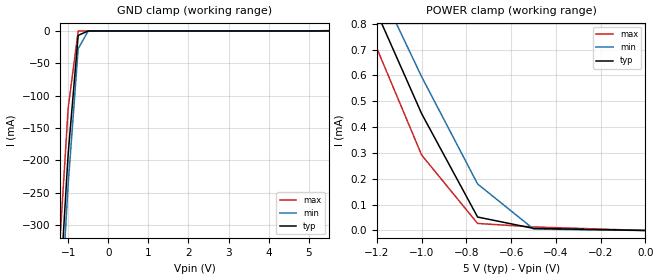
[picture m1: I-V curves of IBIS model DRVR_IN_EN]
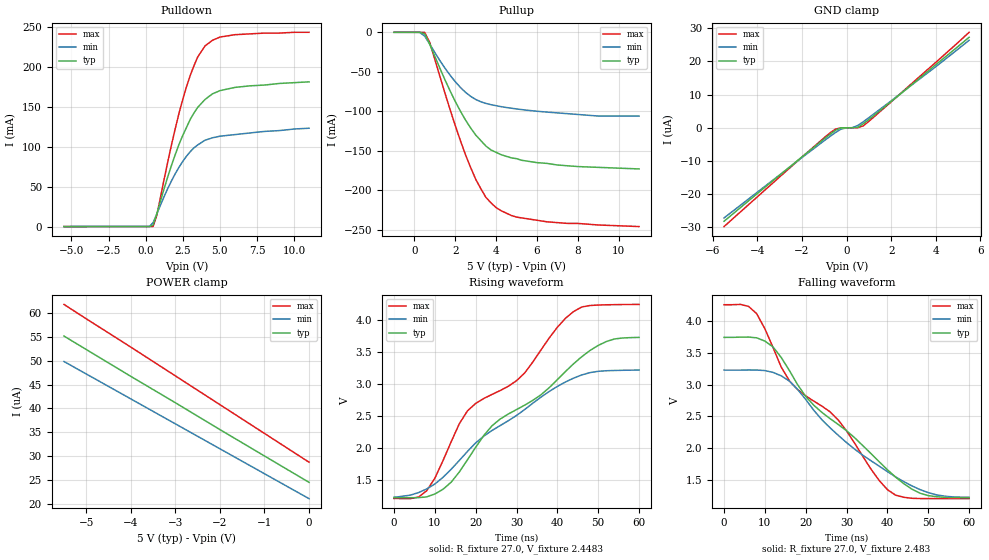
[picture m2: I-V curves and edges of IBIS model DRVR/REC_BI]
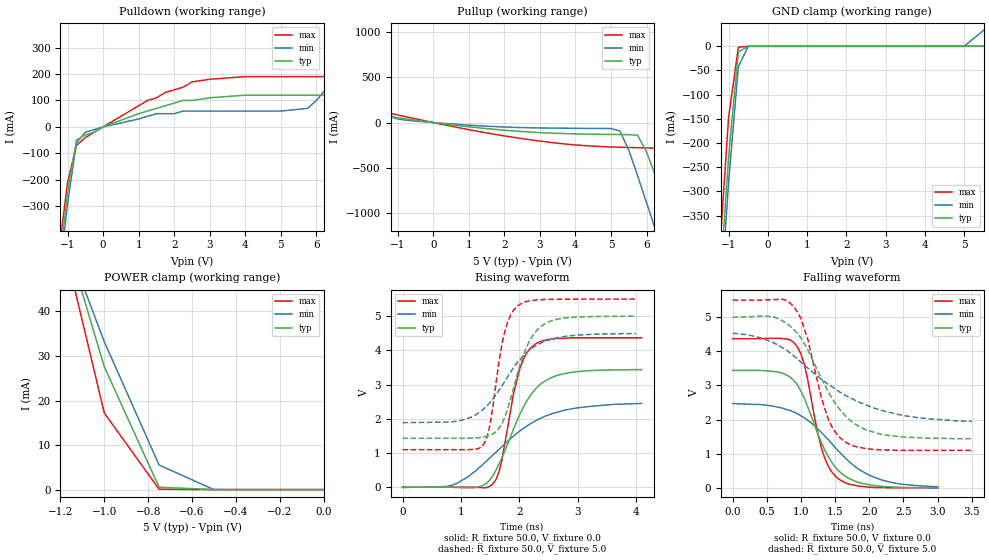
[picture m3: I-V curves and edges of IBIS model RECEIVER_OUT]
|   Texas Instruments Incorporated
|   Data Transmissions Products
|   IBIS Model for SN65HVD24
|   8D SOIC Package
[IBIS Ver]   3.2
[Comment char]   |_char
[File name]   sllc159a.ibs
[File Rev]   1.0
[Date]   19Jun03
[Source]   File originated at Texas Instruments Incorporated.
   Data Transmission Products Group.
[Notes]
[Disclaimer]
(C) Copyright Texas Instruments Incorporated 2003
   All rights reserved
  Texas Instruments Incorporated hereby grants the user of this IBIS
model a non-exclusive, nontransferable license to use this IBIS model
under the following terms.  Before using this IBIS model, the user
should read this license.  If the user does not accept these terms,
the IBIS model should be returned to Texas Instruments within 30 days.
  The user is granted this license only to use the IBIS model and
is not granted rights to sell, load, rent, lease or license the IBIS
model in whole or in part, or in modified form to anyone other than
user.  User may modify the IBIS model to suit its specific applications
but rights to derivative works and such modifications shall belong to
Texas Instruments.
  This IBIS model is provided on an "AS IS" basis and Texas Instruments
makes absolutely no warranty with respect to the information contained
herein.  TEXAS INSTRUMENTS DISCLAIMS AND CUSTOMER WAIVES ALL WARRANTIES,
EXPRESS OR IMPLIED, INCLUDING WARRANTIES OF MERCHANTABILITY OR FITNESS
FOR A PARTICULAR PURPOSE. The entire risk as to quality and performance
is with the Customer. ACCORDINGLY, IN NO EVENT SHALL THE COMPANY BE LIABLE
FOR ANY DAMAGES, WHETHER IN CONTRACT OR TORT,INCLUDING ANY LOST PROFITS
OR OTHER INCIDENTAL, CONSEQUENTIAL, EXEMPLARY, OR PUNITIVE DAMAGES ARISING
OUT OF THE USE OR APPLICATION OF THE IBIS model provided in this package.
Further, Texas Instruments reserves the right to discontinue or make changes
without notice to any product herein to improve reliability, function, or
design. Texas Instruments does not convey any license under patent rights
or any other intellectual property rights, including those of third parties.
Contact Texas Instruments at ATTN:DATA TRANSMISSIONS
[Copyright]   Copyright 2003, Texas Instruments, All Rights Reserved
[Component]   HVD24D
[Manufacturer]  Texas Instruments Incorporated
[Package]
|   typ   min   max
R_pkg   0.055   0.034   0.067
L_pkg   1.795nH   1.699nH   1.914nH
C_pkg   0.299pF   0.278pF   0.311pF
[Pin]   signal_name   model_name   R_pin   L_pin   C_pin
1   R   RECEIVER_OUT   0.067   1.914n   0.278p
2   RE   DRVR_IN_EN   0.062   1.816n   0.301p
3   DE   DRVR_IN_EN   0.053   1.699n   0.298p
4   D   DRVR_IN_EN   0.067   1.907n   0.278p
5   GND   GND   0.034   1.704n   0.311p
6   A   DRVR/REC_BI   0.061   1.808n   0.310p
7   B   DRVR/REC_BI   0.062   1.817n   0.302p
8   VCC   POWER   0.034   1.716n   0.311p
[Diff_pin]   inv_pin   vdiff   tdelay_typ   tdelay_min   tdelay_max
| The 'A' pin is Diff_pin and the 'B' pin is the inv_pin
6   7   0.200   0 0 0
| Models and submodels in the file (3): DRVR_IN_EN (Input), DRVR/REC_BI (I/O), RECEIVER_OUT (3-state)
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|   Driver Input / Receiver Enable Model
[Model]   DRVR_IN_EN
Model_type   Input
|Signals   D,DE,RE
Vinh = 2.0
Vinl = 0.8
|   typ   min   max
C_comp   1.0pF   NA   NA
|   typ   min   max
[Temperature Range]   25.0   -40   125
[Voltage range]   5.0V   4.5V   5.5V
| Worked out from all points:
|   GND clamp passes 1 mA (typ) near -0.54 V on its own axis
|   POWER clamp passes 1 mA (typ) near -1.28 V on its own axis
[GND_clamp]
|   Voltage   I(typ)   I(min)   I(max)
-5.5V     -4.7A      -4.83A     -4.52A
-2V       -1.22A     -1.29A     -1.12A
-1V       -190mA     -237mA     -119mA
-750mV    -6.83mA    -27.3mA    -170uA
-500mV    -28.3uA    -38.2uA    -58.3uA
5.5V      8.09uA     595uA      14.3pA
[Power_clamp]
| Note that the[POWER_clamp]voltage table is referenced to Vcc
| and is calculated using Vtable=Vcc - Vmeasured.
|   Voltage   I(typ)   I(min)   I(max)
-5.5V     9.83mA     9.25mA     10.5mA
-1.25V    941uA      1.05mA     808uA
-1V       452uA      595uA      292uA
-750mV    52uA       180uA      27.1uA
-500mV    8.09uA     5.88uA     13.7uA
0V        0A         0A         0A
|   Driver Output / Receiver Input Model
[Model]   DRVR/REC_BI
Model_type   I/O
| Signals   A,B
Vinl = 0.9V
Vinh = 2.8V
Vmeas = 1.7V   |Reference voltage for timing measurements
Cref = 50pF   |Timing specification test load capacitance value
Rref = 54   |Note: 54 Ohm load; single-ended configuration
|   Timing specification test load voltage
| variable   typ   min   max
C_comp   1.0pF   NA   NA
|   typ   min   max
[Temperature Range]   25.0   -40   85
[Voltage range]   5.0V   4.5V   5.5V
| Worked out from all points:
|   slope of the pulldown table from 0 to 0.75 V, typ, clamps not added: 47.1 ohm
|   slope of the pullup table from 0 to 0.75 V, typ, clamps not added: 49.5 ohm
|   rising waveform, R_fixture 27.0, V_fixture 2.4483: 20-80 % time 25.5ns typ, 23.2ns min, 25ns max; typ from 1.23 V to 3.73 V
|   falling waveform, R_fixture 27.0, V_fixture 2.483: 20-80 % time 23.1ns typ, 20.9ns min, 23ns max; typ from 3.74 V to 1.23 V
[Pulldown]
|   Voltage   I(typ)   I(min)   I(max)
-5.5V     -47.3uA    -37.5uA    -52.8uA
250mV     -13.8uA    29.6uA     -17uA
500mV     1.9mA      4.84mA     48.4uA
750mV     15.9mA     15.6mA     13.8mA
1.75V     77.1mA     57.5mA     103mA
2.5V      114mA      81.5mA     159mA
3.25V     142mA      98.4mA     201mA
3.5V      149mA      102mA      212mA
4V        159mA      108mA      226mA
5V        170mA      113mA      237mA
6V        174mA      115mA      240mA
11V       181mA      123mA      243mA
[Pullup]
|   Voltage   I(typ)   I(min)   I(max)
| Note that the[Pullup]voltage table is referenced to Vcc
| and is calculated using Vtable=Vcc - Vmeasured.
-1V       78uA       65.4uA     90.8uA
250mV     57.2uA     6.09uA     70uA
500mV     -1.82mA    -4.63mA    1.15uA
750mV     -15.1mA    -14.9mA    -12.9mA
1.75V     -74.3mA    -54.4mA    -98.1mA
2.25V     -99.7mA    -69.7mA    -137mA
2.75V     -121mA     -81mA      -171mA
3.5V      -144mA     -90mA      -209mA
4V        -152mA     -92.9mA    -222mA
5V        -160mA     -97mA      -234mA
6.5V      -166mA     -101mA     -240mA
11V       -173mA     -106mA     -246mA
[GND_clamp]
|   Voltage   I(typ)   I(min)   I(max)
| Outputs in High Impedance (off)
-5.5V     -28.2uA    -27.2uA    -29.8uA
-2V       -8.77uA    -8.98uA    -8.83uA
-750mV    -2.01uA    -2.64uA    -1.6uA
-500mV    -761nA     -1.45uA    -411nA
-250mV    -19.5nA    -417nA     -9.75nA
0V        -3.7nA     -3.55nA    -3.96nA
250mV     -3.11nA    22.2nA     -3.43nA
500mV     129nA      679nA      -2.68nA
750mV     1.2uA      1.82uA     578nA
4V        19uA       18.4uA     19.7uA
5.5V      27.3uA     26.4uA     28.8uA
[POWER_clamp]
|   Voltage   I(typ)   I(min)   I(max)
| Note that the [POWER_clamp] voltage table is referenced to Vcc
| and is calculated using Vtable = Vcc - Vmeasured.
| Outputs in Tri-state.
-5.5V     55.1uA     49.8uA     61.7uA
-5V       52.3uA     47.2uA     58.7uA
-4V       46.7uA     42uA       52.8uA
-3V       41.2uA     36.8uA     46.8uA
-2V       35.6uA     31.6uA     40.8uA
-1V       30.1uA     26.4uA     34.8uA
0V        24.6uA     21.2uA     28.8uA
[Ramp]
|   typ   min   max
dV/dt_r   1.50V/25.4ns   1.20V/22.6ns   1.82V/25.0ns
dV/dt_f   1.51V/23.1ns   1.20V/20.9ns   1.82V/23.0ns
R_load = 27ohm | Note: The measurement is on a single-ended configuration
|   with 54ohm line-to-line.
[Rising Waveform]
R_fixture = 27.0
V_fixture = 2.4483
V_fixture_min = 2.227
V_fixture_max = 2.73
C_fixture = 0p
L_fixture = 0n
|   V(typ)   V(min)   V(max)
0s        1.226V     1.228V     1.211V
8ns       1.236V     1.36V      1.331V
12ns      1.355V     1.542V     1.803V
18ns      1.817V     1.948V     2.582V
24ns      2.348V     2.274V     2.838V
30ns      2.601V     2.509V     3.052V
36ns      2.833V     2.796V     3.535V
44ns      3.319V     3.093V     4.135V
52ns      3.665V     3.208V     4.239V
60ns      3.729V     3.219V     4.245V
[Falling Waveform]
R_fixture = 27.0
V_fixture = 2.483
V_fixture_min = 2.227
V_fixture_max = 2.73
C_fixture = 0p
L_fixture = 0n
|   V(typ)   V(min)   V(max)
0s        3.74V      3.227V     4.252V
6ns       3.745V     3.229V     4.226V
8ns       3.733V     3.228V     4.111V
12ns      3.59V      3.191V     3.582V
16ns      3.221V     3.055V     3.06V
22ns      2.675V     2.595V     2.74V
28ns      2.373V     2.203V     2.443V
40ns      1.665V     1.636V     1.353V
48ns      1.297V     1.354V     1.214V
60ns      1.229V     1.232V     1.212V
|   Receiver Output Model
[Model]   RECEIVER_OUT
Model_type   3-state
| Signals   R
Vmeas = 2.2V   |Reference voltage for timing measurements
Cref = 15pF   |Timing specification test load capacitance value
Vref = 0   |Timing specification test load voltage; GND
| variable   typ   min   max
C_comp   1.0pF   NA   NA
|   typ   min   max
[Temperature Range]   25.0   -40   85
[Voltage range]   5.0V   4.5V   5.5V
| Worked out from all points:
|   slope of the pulldown table from 0 to 0.75 V, typ, clamps not added: 20 ohm
|   slope of the pullup table from 0 to 0.75 V, typ, clamps not added: 21 ohm
|   GND clamp passes 1 mA (typ) near -0.52 V on its own axis
|   POWER clamp passes 1 mA (typ) near -0.75 V on its own axis
|   rising waveform, R_fixture 50.0, V_fixture 0.0: 20-80 % time 566ps typ, 1.04ns min, 306ps max; typ from 0 V to 3.44 V
|   falling waveform, R_fixture 50.0, V_fixture 0.0: 20-80 % time 454ps typ, 770ps min, 285ps max; typ from 3.44 V to 0 V
|   rising waveform, R_fixture 50.0, V_fixture 5.0: 20-80 % time 409ps typ, 689ps min, 252ps max; typ from 1.43 V to 5 V
|   falling waveform, R_fixture 50.0, V_fixture 5.0: 20-80 % time 602ps typ, 1.1ns min, 351ps max; typ from 5 V to 1.44 V
[Pulldown]
|   Voltage   I(typ)   I(min)   I(max)
-5.5V     -5.53A     -5.49A     -5.57A
-1.25V    -540mA     -580mA     -480mA
-1V       -250mA     -290mA     -210mA
-750mV    -50mA      -60mA      -70mA
-500mV    -30mA      -20mA      -40mA
1.25V     60mA       40mA       100mA
2.5V      100mA      60mA       170mA
5.75V     120mA      70mA       190mA
6.5V      130mA      170mA      190mA
7.25V     250mA      270mA      200mA
8V        380mA      380mA      360mA
11V       920mA      800mA      1.05A
[Pullup]
|   Voltage   I(typ)   I(min)   I(max)
| Note that the[Pullup]voltage table is referenced to Vcc
| and is calculated using Vtable=Vcc - Vmeasured.
-5.5V     831mA      660mA      1.05A
-1.5V     116mA      101mA      135mA
-750mV    38.6mA     25.2mA     62.6mA
1.5V      -66.6mA    -39.9mA    -114mA
5.25V     -132mA     -93mA      -272mA
5.75V     -140mA     -586mA     -277mA
6V        -324mA     -882mA     -279mA
6.25V     -583mA     -1.18A     -282mA
6.5V      -849mA     -1.47A     -402mA
7V        -1.44A     -2.06A     -909mA
8V        -2.62A     -3.21A     -1.99A
11V       -6.03A     -6.64A     -5.58A
[GND_clamp]
|   Voltage   I(typ)   I(min)   I(max)
| Outputs in High Impedance (off)
-5.5V     -5.53A     -5.49A     -5.57A
-1.25V    -531mA     -579mA     -452mA
-1V       -230mA     -282mA     -148mA
-750mV    -11.8mA    -42mA      -2.02mA
-500mV    -7.54uA    -155uA     -41.3uA
5V        0A         5.88uA     -7.45nA
5.5V      22.4nA     33.2mA     -7.45nA
[POWER_clamp]
|   Voltage   I(typ)   I(min)   I(max)
| Note that the [POWER_clamp] voltage table is referenced to Vcc
| and is calculated using Vtable = Vcc - Vmeasured.
| Outputs in Tri-state.
-5.5V     845mA      659mA      1.05A
-1.25V    68.8mA     65.7mA     68.8mA
-1V       27.6mA     33.2mA     17.2mA
-750mV    537uA      5.52mA     88.4uA
-500mV    22.4nA     5.88uA     0A
0V        0A         0A         -7.45nA
[Ramp]
|   typ   min   max
dV/dt_r   2.06V/563ns   1.47V/1038ps   2.62V/306ps
dV/dt_f   2.14V/599ps   1.55V/1103ps   2.64V/346ps
R_load = 50
[Rising Waveform]
R_fixture = 50.0
V_fixture = 0.0
C_fixture = 0p
L_fixture = 0n
|   V(typ)   V(min)   V(max)
0s        0V         -10mV      0V
900ps     -10mV      90mV       0V
1.35ns    30mV       620mV      -10mV
1.55ns    340mV      940mV      100mV
1.7ns     840mV      1.18V      760mV
1.9ns     1.69V      1.49V      2.71V
2ns       2.09V      1.63V      3.41V
2.3ns     2.91V      1.96V      4.21V
2.9ns     3.36V      2.29V      4.37V
4.1ns     3.44V      2.45V      4.37V
[Falling Waveform]
R_fixture = 50.0
V_fixture = 0.0
C_fixture = 0p
L_fixture = 0n
|   V(typ)   V(min)   V(max)
0s        3.44V      2.47V      4.37V
700ps     3.38V      2.35V      4.38V
950ps     3.01V      2.17V      4.12V
1.05ns    2.62V      2.05V      3.61V
1.3ns     1.32V      1.62V      1.16V
1.4ns     910mV      1.41V      630mV
1.55ns    500mV      1.07V      260mV
1.8ns     190mV      610mV      70mV
2.1ns     60mV       290mV      10mV
3ns       0V         30mV       0V
[Rising Waveform]
R_fixture = 50.0
V_fixture = 5.0
V_fixture_min = 4.5
V_fixture_max = 5.5
C_fixture = 0p
L_fixture = 0n
|   V(typ)   V(min)   V(max)
0s        1.43V      1.887V     1.097V
950ps     1.428V     1.938V     1.096V
1.4ns     1.472V     2.302V     1.276V
1.5ns     1.519V     2.481V     1.827V
1.65ns    1.709V     2.822V     3.631V
1.75ns    2.037V     3.084V     4.53V
2ns       3.497V     3.713V     5.336V
2.2ns     4.345V     4.039V     5.456V
2.5ns     4.831V     4.303V     5.492V
4ns       4.999V     4.493V     5.5V
[Falling Waveform]
R_fixture = 50.0
V_fixture = 5.0
V_fixture_min = 4.5
V_fixture_max = 5.5
C_fixture = 0p
L_fixture = 0n
|   V(typ)   V(min)   V(max)
0s        5V         4.53V      5.5V
600ps     5.01V      4.25V      5.52V
900ps     4.63V      3.86V      5.29V
1ns       4.39V      3.68V      4.96V
1.1ns     4.04V      3.51V      4.35V
1.3ns     3.2V       3.18V      2.63V
1.4ns     2.81V      3.03V      2.01V
1.65ns    2.11V      2.71V      1.34V
2.2ns     1.56V      2.26V      1.11V
3.5ns     1.44V      1.95V      1.1V
